(* Logix 5000 AddOnInstructionDefinition export MAC_G3_MAFR; software revision 37.00 *)

TYPE JVL_AXIS_MAC_G3 :   // Drive Data
STRUCT
   ActualMode : DINT;   // actual Mode
   ActualPosition : REAL;   // P_IST
   ActualVelocity : REAL;   // V_IST(16)
   ActualTorque : REAL;   // ACTUAL_TORQUE
   AxisStatusError : JVL_MAC_Status_Error;   // Holds an indication of which error that is detected
   Home_Mode : DINT;   // Homemode
   RequestedMode : DINT;   // requested Mode
   RequestedPosition : REAL;   // P_SOLL
   RequestedVelocity : REAL;   // V_SOLL
   RequestedAcceleration : REAL;   // A_SOLL
   GeneralCommand : DINT;
   CommandTorque : REAL;   // Requested Torque, T_SOLL
   ZeroSearchVelocity : REAL;   // Homing velocity
   ZeroSearchPosition : REAL;   // Homing position
   ZeroSearchTorque : DINT;   // Homing torque setpoint threshold value
   ZeroSearchTThreshold : DINT;   // Threshold for torque zerosearch trigger, usually 20% lower than running torque
   TravelConst : REAL;   // Factor to multiply P_IST and P_SOLL for scaling
   VelConst : REAL;   // Factor to multiply V_SOLL and V_IST to get scaled velocity value
   HomingType : DINT;   // Holds the reqested homingtype
   LoadFactor : DINT;   // Inertia ratio motor/load
   MotorType : DINT;   // MotorType configured. 0=No Selection 1=MAC50-141-A/K (old) 2=MAC50-141-F (new), MAC400, 402, 1500, 3000, 4500 (All Encoder variations) 3=MAC800 with incremental encoder 4=MAC800 with abs. encoder
   Configured : DINT;
   MSG_OutValue : DINT;   // Used in exp. output message to the motor
   MSG_InValue : DINT;   // Used in Exp. output message, to get value from motor
   MSG_OutInstance : DINT;   // Registernumber
   MSG_InInstance : DINT;   // Registernummer
   V_SOLL_CountsPerSample : REAL;
   A_SOLL_CountsPerSample2 : REAL;
   AOI_Type : DINT;   // MAC_Disable = 1, MAC_Home = 2, MAC_Jog = 3, MAC_Position = 4, MAC_Reset = 5, MAC_Stop = 6
   Position_AppType : REAL;   // calculated Position by Application Type
   MSG_Out_Execute : BOOL;   // Enable MSG_Out
   MSG_In_Execute : BOOL;   // Enable MSG_In
   ErrorReset : BOOL;
   MSG_Out_Busy : BOOL;
   MSG_In_Busy : BOOL;
   MSG_Out_Done : BOOL;
   MSG_In_Done : BOOL;
END_STRUCT
END_TYPE

TYPE JVL_MAC_Status_Error :   // Axis Faults Status
STRUCT
   Error : BOOL;
   InitialisationError : BOOL;
   FlashMemoryError : BOOL;
   STOError : BOOL;
   NotUsed_2 : BOOL;
   NotUsed_3 : BOOL;
   OUT1 : BOOL;
   OUT2 : BOOL;
   NotUsed : BOOL;
   ControlVoltageError : BOOL;
   HomingDone : BOOL;
   MotorSupplyDetected : BOOL;
   MotorLocked : BOOL;
   CommsError : BOOL;
   CurrentLoopError : BOOL;
   ModbusSlaveError : BOOL;
   TemperatureError : BOOL;
   UndervoltageError : BOOL;
   UndervoltageDetect : BOOL;
   OvervoltageError : BOOL;
   OvercurrentError : BOOL;
   OverspeedError : BOOL;
   AllowExceedingOfSoftwareLimits : BOOL;
   EncoderError : BOOL;
   I2TError : BOOL;
   FollowingError : BOOL;
   FunctionError : BOOL;
   BreakingResistorOverTempError : BOOL;
   InPosition : BOOL;
   Accelerating : BOOL;
   Decelerating : BOOL;
   SoftwareLimitExceeded : BOOL;
END_STRUCT
END_TYPE

ADD_ON_INSTRUCTION MAC_G3_MAFR   (* revision 1.0, ExecuteEnableInFalse *)
VAR_IN_OUT
   AXIS : JVL_AXIS_MAC_G3; {required}
END_VAR
VAR_OUTPUT
   EN : BOOL; {access Read Only, visible}
   CommandAborted : BOOL; {access Read Only}
   DN : BOOL; {access Read Only, visible}
   ER : BOOL; {visible}
END_VAR
VAR
   State : INT; {access None}
   ExecuteStart : BOOL; {access None}
   AOI_Type : DINT; {access None}
END_VAR

ROUTINE EnableInFalse   (* structured text *)
   State := 0;
   ExecuteStart:=0;
   	//REGION STATUS SIGNALS
   
   	    DN := State = 30;
   	    CommandAborted := State = 80;
   	    EN := EnableOut;
   	    ER:= AXIS.AxisStatusError.Error;
   	//END_REGION
   
END_ROUTINE

ROUTINE Logic   (* structured text *)
   	(*********************
   		Error Reset
   	**********************)
   
   	//REGION CAPTURE EDGES
   	    if EnableIn and not ExecuteStart then
   	    	ExecuteStart:=1;
   		//elsif not EnableIn then
   			//ExecuteStart:=0;
   		end_if;
   
   	//END_REGION
   
   	//REGION STATE CHANGES
   
   	    //Re-trigger sequence from start on rising edge
   	    //Command aborted
   	    IF AXIS.AOI_Type <> AOI_Type AND
   	        State <> 0 AND
   	        State <> 90 AND
   	        State <> 30 AND
   	        State <> 80
   	    THEN
   	        State := 80;
   	    END_IF;
   
   
   	//END_REGION
   
   	//REGION STATE MACHINE
   
   	    CASE State OF
   
   	        0:
   	            IF ExecuteStart THEN
   					AOI_Type:= 5;
   					AXIS.AOI_Type:= 5;
   	                AXIS.GeneralCommand := 16#0;
   	                State := 10;
   	            END_IF;
   
   	        10:
   	            AXIS.RequestedMode := 0;
   	            AXIS.RequestedAcceleration := 0;
   	            AXIS.RequestedPosition := 0;
   	            AXIS.RequestedVelocity := 0;
   	            AXIS.GeneralCommand := 16#10000E1;
   	            IF NOT AXIS.AxisStatusError.Error and AXIS.MotorType<>1 THEN
   	                State := 20;
   
   	            END_IF;
   
   
   	        20:
   	            AXIS.GeneralCommand := 16#0;
   	            State := 30;
   
   	        30:        //reset complete, reset to idle by setting execute false
   	            ;
   
   	        80:     //Aborted by other command before completion
   	            ;
   
   	        90:       //Error while disabling, reset to idle by setting execute false
   	            ;
   
   	        ELSE
   	            ;
   
   	    END_CASE;
   
   	//END_REGION
   
   	//REGION STATUS SIGNALS
   
   	    DN := State = 30;
   	    CommandAborted := State = 80;
   	    EN := EnableOut;
   	    ER:= AXIS.AxisStatusError.Error;
   	//END_REGION
   
END_ROUTINE
END_ADD_ON_INSTRUCTION

ADD_ON_INSTRUCTION MAC_G3_MAH   (* revision 1.0, ExecuteEnableInFalse *)
VAR_IN_OUT
   Axis : JVL_AXIS_MAC_G3; {required}
END_VAR
VAR_OUTPUT
   CommandAborted : BOOL; {access Read Only}
   EN : BOOL; {access Read Only, visible}   // Enable Bit - The EN bit stays Set until the Process is Complete and the rung goes False
   DN : BOOL; {access Read Only, visible}   // Done Bit - The Done bit is Set if the Instruction Executed without Errors
   ER : BOOL; {access Read Only, visible}   // Error Bit - An Error Happened
   IP : BOOL; {access Read Only, visible}   // In Progress Bit - The In Progress bit is Set While the Axis is Moving
   PC : BOOL; {access Read Only, visible}   // Process Complete, Motion has stopped
END_VAR
VAR_INPUT
   Mode : INT; {required}   // 0 = set Encoder, 1 = Homing on Sensor, 2 = Homing on Block
   Position : REAL; {required}   // Scaled Position after setting Encoder, with Mode = 0
   Speed : REAL; {required}   // Scaled velocity
   Acceleration : REAL; {required}   // in RPM/s
   Offset : REAL; {required}   // scaled Position after Homing, with Mode = 1 or 2
   TorqueLimit : REAL; {required}   // Homing Torque in %
END_VAR
VAR
   State : INT; {access None}
   ActiveMode : INT; {access None}
   Mode0State : INT; {access None}
   Mode1State : INT; {access None}
   Mode2State : INT; {access None}
   Mode3State : INT; {access None}
   ActivePosition : DINT; {access None}
   ActiveVelocity : DINT; {access None}
   ActiveAcceleration : REAL; {access None}
   ActiveTorqueLimit : REAL; {access None}
   ExecuteStart : BOOL; {access None}
   AOI_Type : DINT; {access None}
   ActiveDeceleration : DINT; {access None}
   Ton_wait : FBD_TIMER; {access None}
   ActiveOffset : DINT; {access None}
END_VAR

ROUTINE EnableInFalse   (* structured text *)
   State := 0;
   ExecuteStart:=0;
   	//REGION STATUS SIGNALS
   
   	    DN := State = 30;
   	    CommandAborted := State = 80;
   	    ER := State = 90;
   	    IP := State <> 0 AND NOT DN AND NOT ER AND NOT CommandAborted;
   	    EN := EnableOut;
   		PC := State = 30;
   	//END_REGION
END_ROUTINE

ROUTINE Logic   (* structured text *)
   	//REGION CAPTURE EDGES
   	    if EnableIn and not ExecuteStart then
   	    	ExecuteStart:=1;
               Axis.MSG_Out_Execute := 0;
               Axis.MSG_In_Execute := 0;
   			Ton_wait.TimerEnable:=0;
   			Ton_wait.Reset:=0;
   		elsif not EnableIn then
   			ExecuteStart:=0;
   		end_if;
   
   	//END_REGION
   	//Timer
   	TONR(Ton_wait);
   
   	//REGION STATE CHANGES
   
   	    //Re-trigger sequence from start on rising edge
   
   
   	    //Command aborted
   	    IF Axis.AOI_Type <> AOI_Type AND
   	        State <> 0 AND
   	        State <> 90 AND
   	        State <> 30 AND
   	        State <> 80
   	    THEN
   	        State := 80;
   	    END_IF;
   
   
   	    //Error if motor error while executing
   	    IF Axis.AxisStatusError.Error AND
   	        State <> 0 AND
   	        State <> 90 AND
   	        State <> 30 AND
   	        State <> 80
   	    THEN
   	        State := 90;
   	    END_IF;
   	//END_REGION
   
   	//REGION STATE MACHINE
   
   
   
   	    CASE State OF
   
   	        0:
   	            //Reset static values
   	            ActiveMode := 0;
   	            ActivePosition := 0;
   	            ActiveVelocity := 0;
   				ActiveAcceleration := 0;
   	            ActiveDeceleration := 0;
   				ActiveTorqueLimit := 0;
   	            ActiveOffset := 0;
   	            //Reset mode states
   	            Mode0State := 0;
   	            Mode1State := 0;
   	            Mode2State := 0;
   	            Mode3State := 0;
   
   	            IF ExecuteStart THEN
   					//
   					AOI_Type:= 2;
   					Axis.AOI_Type:= 2;
   	                //
   					Axis.GeneralCommand := 0;
   	                ActiveMode := Mode;
   	                ActivePosition := Position * Axis.TravelConst;
   	                ActiveVelocity := (Speed) * Axis.VelConst;// * Axis.Device.Config.V_SOLL_CountsPerSample);
   	                ActiveAcceleration := ABS(Acceleration) * Axis.A_SOLL_CountsPerSample2;
   	                //set Acceleration always >=1
   	                IF ActiveAcceleration < 1 THEN
   	                    ActiveAcceleration := 1;
   	                END_IF;
   
   	                ActiveTorqueLimit := TorqueLimit * 3.41;//1024=300%;341=100%
   	                ActiveOffset := Offset * Axis.TravelConst;
   
   
   	                State := 10;
   	            END_IF;
   
   	        10:
   	            // change to velocity mode with zero setpoint to ensure motor does not run off to current position when homed
   	            IF ActiveAcceleration < 1 THEN
   	                Axis.RequestedAcceleration := 1;
   	            ELSE
   	                Axis.RequestedAcceleration := ActiveAcceleration;
   
   	            END_IF;
   	            Axis.RequestedVelocity := 0;
   	            Axis.RequestedMode := 1;
   	            // change position setpoint to new home position
   	            Axis.RequestedPosition := ActivePosition;
   	            // reset register trigger
   	            Axis.MSG_Out_Execute := 0;
   	            Axis.MSG_In_Execute := 0;
   	            // start homing
   	            State := 20;
   
   	        20:
   	            CASE ActiveMode OF
   
   	                0:  // Set Home Position
   	                    CASE Mode0State OF
   	                        0:
   	                            if Axis.MotorType=1 then
   									Axis.MSG_OutInstance := 163;
   								else
   									Axis.MSG_OutInstance := 4;
   								end_if;
   	                            Axis.MSG_OutValue:=ActivePosition;
   	                            Axis.MSG_Out_Execute := 1;
   	                            Axis.GeneralCommand := 16#0;
   	                            IF Axis.MSG_Out_Busy AND NOT Axis.MSG_Out_Done THEN
   	                                Mode0State := 10;
   	                            END_IF;
   	                        10:
   	                            IF Axis.MSG_Out_Done THEN
   	                                Axis.MSG_Out_Execute := 0;
   	                                Mode0State := 20;
   	                            END_IF;
   	                        20:
   	                            Axis.GeneralCommand := 16#10000F7;
   	                            IF ABS(Axis.ActualPosition - ActivePosition) < 50.0 THEN
   	                                Mode0State := 30;
   	                            END_IF;
   	                        30:
   	                            Axis.GeneralCommand := 16#0;
   	                            Mode0State := 50;
   	                        50:
   	                            State := 30;
   	                        ELSE
   	                            State := 90;
   	                    END_CASE;
   
   	                1:  // Home to Sensor (type 2, bidirectional)
   	                    CASE Mode1State OF
   	                       0:
   	                            // reset hominging done bit old MAC050-141A/K
   	                                IF Axis.MotorType <> 1 THEN
   	                                    Mode1State := 10;
   	                                ELSE
   		                            Axis.MSG_OutInstance := 168;
   		                            Axis.MSG_OutValue := 0;
   		                            Axis.MSG_Out_Execute := 1;
   			                            IF Axis.MSG_Out_Busy THEN
   			                                Mode1State := 5;
   			                            END_IF;
   	                                END_IF;
   	                        5:
   	                            //Ton_Wait(IN := Reg.Done,PT := t#1s);
   	                            IF Axis.MSG_Out_Done THEN
   	                                Axis.MSG_Out_Execute := 0;
   	                                Mode1State := 10;
   	                            END_IF;
   	                       10:
   	                            //Home to Sensor (type 2);set homemode=3584
   	                            Axis.MSG_OutInstance := 42;
   	                            Axis.MSG_OutValue:=3584;
   
   	                            Axis.MSG_Out_Execute := 1;
   	                            IF Axis.MSG_Out_Busy THEN
   	                                Mode1State := 15;
   	                            END_IF;
   	                       15:
   	                            IF Axis.MSG_Out_Done THEN
   	                                Axis.MSG_Out_Execute := 0;
   	                                Mode1State := 20;
   									Axis.AxisStatusError.HomingDone:=0;
   	                            END_IF;
   
   	                       20:
   	                            // set home position offset move distance
   	                            Axis.MSG_OutInstance := 38;
   	                            Axis.MSG_OutValue:=ActiveOffset;
   	                            Axis.MSG_Out_Execute := 1;
   	                            IF Axis.MSG_Out_Busy THEN
   	                                Mode1State := 30;
   	                            END_IF;
   	                        30:
   	                            IF Axis.MSG_Out_Done THEN
   	                                Axis.MSG_Out_Execute := 0;
   	                                Mode1State := 40;
   	                            END_IF;
   	                        40:
   	                            // set homing approach velocity
   	                            Axis.MSG_OutInstance := 40;
   	                            Axis.MSG_OutValue:=ActiveVelocity;// * Axis.Device.Config.V_SOLL_CountsPerSample
   	                            Axis.MSG_Out_Execute := 1;
   	                            IF Axis.MSG_Out_Busy THEN
   	                                Mode1State := 50;
   	                            END_IF;
   	                        50:
   	                            IF Axis.MSG_Out_Done THEN
   	                                Axis.MSG_Out_Execute := 0;
   	                                Mode1State := 60;
   	                            END_IF;
   	                        60:
   	                            // start homing mode
   	                            Axis.RequestedMode := 14;
   								if Axis.MotorType=1 then
   									Axis.RequestedVelocity := ActiveVelocity;
   								end_if;
   	                            if Axis.ActualMode=14 then
   	                            	Mode1State := 70;
   	                            end_if;
   	                        70:
   	                            IF Axis.AxisStatusError.HomingDone AND Axis.MotorType <> 1 THEN
   	                                Axis.RequestedVelocity := 0;
   	                                Axis.RequestedMode := 2;
   	                                Mode1State := 80;
   	                            ELSIF Axis.Home_Mode > 0 AND Axis.MotorType = 1 THEN
   	                                Axis.RequestedVelocity := 0;
   	                                Axis.RequestedMode := 2;
   	                                Mode1State := 80;
   	                            END_IF;
   	                        80:
   	                            State := 30;
   	                        ELSE
   	                            State := 90;
   	                    END_CASE;
   
   	                2:  // Home to Endstop (torque limit)
   	                    CASE Mode2State OF
   	                        0:
   	                            //Home to Endstop (torque limit);set homemode=3072
   								Axis.MSG_OutInstance := 42;
   	                            Axis.MSG_OutValue := 3072;
   	                            Axis.MSG_Out_Execute := 1;
   
   	                            IF Axis.MSG_Out_Busy THEN
   	                                Mode2State := 5;
   	                            END_IF;
   	                        5:
   	                            IF Axis.MSG_Out_Done THEN
   	                                Axis.MSG_Out_Execute := 0;
   	                                Mode2State := 10;
   	                            END_IF;
   	                        10:
   								Axis.MSG_OutInstance := 38;
   	                            Axis.MSG_OutValue := ActiveOffset;
   	                            Axis.MSG_Out_Execute := 1;
   
   	                            IF Axis.MSG_Out_Busy THEN
   	                                Mode2State := 15;
   	                            END_IF;
   	                        15:
   	                            IF Axis.MSG_Out_Done THEN
   	                                Axis.MSG_Out_Execute := 0;
   	                                Mode2State := 20;
   									Axis.AxisStatusError.HomingDone:=0;
   	                            END_IF;
   	                        20:
   								Axis.MSG_OutInstance := 40;
   	                            Axis.MSG_OutValue := ActiveVelocity;// * Axis.Device.Config.V_SOLL_CountsPerSample;
   	                            Axis.MSG_Out_Execute := 1;
   	                            IF Axis.MSG_Out_Busy THEN
   	                                Mode2State := 25;
   	                            END_IF;
   	                        25:
   	                            IF Axis.MSG_Out_Done THEN
   	                                Axis.MSG_Out_Execute := 0;
   	                                IF Axis.MotorType <> 1 THEN
   	                                    Mode2State := 34;
   	                                ELSE
   	                                    Mode2State := 30;
   	                                END_IF;
   	                            END_IF;
   	                        30:
   	                            // reset hominging done bit old MAC050-141A/K
   								Axis.MSG_OutInstance := 168;
   	                            Axis.MSG_OutValue := 0;
   	                            Axis.MSG_Out_Execute := 1;
   
   	                            IF Axis.MSG_Out_Busy THEN
   	                                Mode2State := 32;
   	                            END_IF;
   	                        32:
   
   	                            IF Axis.MSG_Out_Done THEN
   	                                Axis.MSG_Out_Execute := 0;
   	                                Mode2State := 34;
   	                            END_IF;
   	                        34:
   								Axis.MSG_OutInstance := 41;
   	                            Axis.MSG_OutValue := ActiveTorqueLimit;
   	                            Axis.MSG_Out_Execute := 1;
   
   	                            IF Axis.MSG_Out_Busy THEN
   	                                Mode2State := 37;
   	                            END_IF;
   	                        37:
   	                            IF Axis.MSG_Out_Done THEN
   	                                Axis.MSG_Out_Execute := 0;
   	                                Mode2State := 40;
   	                            END_IF;
   	                        40:
   	                            Axis.RequestedMode := 12;
   	                            // homing done-register 42 Homemode bit 16
   								if Axis.MotorType=1 then
   									Axis.RequestedVelocity := ActiveVelocity;
   								end_if;
   	                            if Axis.ActualMode=12 then
   	                            	Mode2State := 45;
   	                            end_if;
   
   	                        45:
   	                            IF Axis.AxisStatusError.HomingDone AND Axis.MotorType <> 1 THEN
   	                                Axis.RequestedVelocity := 0;
   	                                Axis.RequestedMode := 2;
   	                                Mode2State := 60;
   	                            ELSIF Axis.Home_Mode > 0 AND Axis.MotorType = 1 THEN
   	                                Axis.RequestedVelocity := 0;
   	                                Axis.RequestedMode := 2;
   	                                Mode2State := 60;
   	                            END_IF;
   
   	                        60:
   	                            State := 30;
   	                        ELSE
   	                            State := 90;
   	                    END_CASE;
   
   
   
   	            END_CASE;
   
   	        30:        //Home complete, reset to idle by setting execute false
   	            ;
   
   	        80:     //Aborted by other command before completion
   	            ;
   
   	        90:       //Error while disabling, reset to idle by setting execute false
   	            ;
   
   	        ELSE
   	            ;
   
   	    END_CASE;
   
   	//END_REGION
   
   	//REGION STATUS SIGNALS
   
   	    DN := State = 30;
   	    CommandAborted := State = 80;
   	    ER := State = 90;
   	    IP := State <> 0 AND NOT DN AND NOT ER AND NOT CommandAborted;
   	    EN := EnableOut;
   		PC := State = 30;
   	//END_REGION
END_ROUTINE
END_ADD_ON_INSTRUCTION

ADD_ON_INSTRUCTION MAC_G3_MAJ   (* revision 1.0, ExecuteEnableInFalse *)
VAR_IN_OUT
   AXIS : JVL_AXIS_MAC_G3; {required}
END_VAR
VAR_INPUT
   Direction : DINT; {required}   // 0 = CW rotation, 1 = CCW rotation
   Speed : REAL; {required}   // scaled velocity
   Acceleration : REAL := 5000.0; {required}   // in rpm/s
END_VAR
VAR_OUTPUT
   EN : BOOL; {access Read Only, visible}   // Enable Bit - The EN bit stays Set until the Process is Complete and the rung goes False
   DN : BOOL; {access Read Only, visible}   // Done Bit - The Done bit is Set if the Instruction Executed without Errors
   ER : BOOL; {access Read Only, visible}   // Error Bit - An Error Happened
   IP : BOOL; {access Read Only, visible}   // In Progress Bit - The In Progress bit is Set While the Axis is Moving
END_VAR
VAR
   ForwardStart : BOOL; {access None}
   BackwardStart : BOOL; {access None}
   State : INT; {access None}
   ActiveVelocity : REAL; {access None}
   ActiveAcceleration : REAL; {access None}
   AOI_Type : DINT; {access None}
   ActiveDeceleration : REAL; {access None}
END_VAR

ROUTINE EnableInFalse   (* structured text *)
   	//REGION CAPTURE EDGES
   	    if Direction = 0 and EnableIn then
   	    	ForwardStart:=1;
   	    elsif Direction = 1 and EnableIn then
   	    	BackwardStart:=1;
   		elsif not EnableIn then
   	    	ForwardStart:=0;
   	    	BackwardStart:=0;
   		end_if;
   
   	//END_REGION
   
   	//REGION STATE CHANGES
   
   	    //Re-trigger sequence from start on rising edge
   	    //Command aborted
   	    IF AXIS.AOI_Type <> AOI_Type AND
   	        State <> 0 AND
   	        State <> 90 AND
   	        State <> 80
   	    THEN
   	        State := 80;
   	    END_IF;
   
   
   
   	    //Error if motor error while executing
   	    IF AXIS.AxisStatusError.Error AND
   	        State <> 0 AND
   	        State <> 90 AND
   	        State <> 80
   	    THEN
   	        State := 90;
   	    END_IF;
   
   	//END_REGION
   
   	//REGION STATE MACHINE
   
   	    CASE State OF
   
   	        0:
   	            ActiveVelocity := 0;
   	            ActiveAcceleration := 0;
   	            ActiveDeceleration := 0;
   
   	            IF ForwardStart OR BackwardStart THEN
   					DN := 0;
   					AOI_Type:= 3;
   					AXIS.AOI_Type:= 3;
   	                AXIS.RequestedMode:= 1;
   	                ActiveAcceleration := ABS(Acceleration);
   
   	                //set Acceleration always >=1
   	                IF ActiveAcceleration < 1 THEN
   	                    ActiveAcceleration := 1;
   	                END_IF;
   	                IF Direction = 0 THEN
   	                    ActiveVelocity := ABS(Speed) * AXIS.VelConst;// * Axis.Device.Config.V_SOLL_CountsPerSample));
   	                    State := 10;
   	                ELSIF Direction = 1 THEN
   	                    ActiveVelocity := -1.0 * ABS(Speed)* AXIS.VelConst;// * Axis.Device.Config.V_SOLL_CountsPerSample));
   	                    State := 10;
   	                ELSE
   	                    State := 30;
   	                END_IF;
   
   	                State := 10;
   	            END_IF;
   
   	        10:
   	            IF AXIS.ActualMode = 1 THEN
   
   	                AXIS.RequestedAcceleration := ActiveAcceleration;
   	                AXIS.RequestedVelocity := ActiveVelocity;
                       State := 30;
   
   	            END_IF;
   
   	        20:
   	            IF AXIS.ActualMode = 1 THEN
   
   	                IF not EnableIn THEN
   	                    State := 30;
   	                END_IF;
   
   	            ELSE
   	                State := 80;
   	            END_IF;
   
   
   	        30:
   	            AXIS.RequestedMode := 1;
   	            AXIS.RequestedVelocity := 0;
   
   	            State := 40;
   
   	        40:
   	            IF AXIS.ActualMode = 1  THEN
   
   	                //If no motion then stop is complete
   	                IF ABS((AXIS.ActualVelocity)) <= 10.0 AND
   	                    NOT AXIS.AxisStatusError.Accelerating AND
   	                    NOT AXIS.AxisStatusError.Decelerating THEN
   	                    State := 0;
   						DN := 1;
   	                END_IF;
   
   	            ELSE
   	                State := 80;
   	            END_IF;
   
   	        80:     //Aborted by other command before completion
   	            IF NOT EnableIn THEN
   	                State := 0;
   	            END_IF;
   
   	        90:       //Error while jogging, reset to idle by setting jog inputs false
   	            IF NOT EnableIn THEN
   	                State := 0;
   	            END_IF;
   
   	        ELSE
   	            State := 90;
   
   	    END_CASE;
   
   	//END_REGION
   
   	//REGION STATUS SIGNALS
   
   	    EN:=EnableOut;
   						//(State=20 or State = 25) AND
   	                    //  AXIS.AxisStatus.AtVelocity AND
   	                    //  NOT AXIS.AxisStatus.Accelerating AND
   	                    //  NOT AXIS.AxisStatus.Decelerating;
   	    DN := State = 40;
   	    ER := State = 90;
   	    IP := State <> 0 AND NOT ER AND NOT DN;
   
   	//END_REGION
   
END_ROUTINE

ROUTINE Logic   (* structured text *)
   	//REGION CAPTURE EDGES
   	    if Direction = 0 and EnableIn then
   	    	ForwardStart:=1;
   	    elsif Direction = 1 and EnableIn then
   	    	BackwardStart:=1;
   		elsif not EnableIn then
   	    	ForwardStart:=0;
   	    	BackwardStart:=0;
   		end_if;
   
   	//END_REGION
   
   	//REGION STATE CHANGES
   
   	    //Re-trigger sequence from start on rising edge
   	    //Command aborted
   	    IF AXIS.AOI_Type <> AOI_Type AND
   	        State <> 0 AND
   	        State <> 90 AND
   	        State <> 80
   	    THEN
   	        State := 80;
   	    END_IF;
   
   
   
   	    //Error if motor error while executing
   	    IF AXIS.AxisStatusError.Error AND
   	        State <> 0 AND
   	        State <> 90 AND
   	        State <> 80
   	    THEN
   	        State := 90;
   	    END_IF;
   
   	//END_REGION
   
   	//REGION STATE MACHINE
   
   	    CASE State OF
   
   	        0:
   	            ActiveVelocity := 0;
   	            ActiveAcceleration := 0;
   	            ActiveDeceleration := 0;
   
   	            IF ForwardStart OR BackwardStart THEN
   					DN := 0;
   					AOI_Type:= 3;
   					AXIS.AOI_Type:= 3;
   	                AXIS.RequestedMode:= 1;
   	                ActiveAcceleration := ABS(Acceleration)* AXIS.A_SOLL_CountsPerSample2;
   	                //set Acceleration always >=1
   	                IF ActiveAcceleration < 1 THEN
   	                    ActiveAcceleration := 1;
   	                END_IF;
   	                IF Direction = 0 THEN
   	                    ActiveVelocity := ABS(Speed) * AXIS.VelConst;// * Axis.Device.Config.V_SOLL_CountsPerSample));
   	                    State := 10;
   	                ELSIF Direction = 1 THEN
   	                    ActiveVelocity := -1.0 * ABS(Speed)* AXIS.VelConst;// * Axis.Device.Config.V_SOLL_CountsPerSample));
   	                    State := 10;
   	                ELSE
   	                    State := 30;
   	                END_IF;
   
   	                State := 10;
   	            END_IF;
   
   	        10:
   	            IF AXIS.ActualMode = 1 THEN
   
   	                AXIS.RequestedAcceleration := ActiveAcceleration;
   	                AXIS.RequestedVelocity := ActiveVelocity;
   	                IF not EnableIn THEN
   	                    State := 30;
   	                END_IF;
   
   	            END_IF;
   
   	        20:
   	            IF AXIS.ActualMode = 1 THEN
   
   	                IF not EnableIn THEN
   	                    State := 30;
   	                END_IF;
   
   	            ELSE
   	                State := 80;
   	            END_IF;
   
   
   	        30:
   	            AXIS.RequestedMode := 1;
   	            AXIS.RequestedVelocity := 0;
   
   	            State := 40;
   
   	        40:
   	            IF AXIS.ActualMode = 1  THEN
   
   	                //If no motion then stop is complete
   	                IF ABS((AXIS.ActualVelocity)) <= 10.0 AND
   	                    NOT AXIS.AxisStatusError.Accelerating AND
   	                    NOT AXIS.AxisStatusError.Decelerating THEN
   	                    State := 0;
   						DN := 1;
   	                END_IF;
   
   	            ELSE
   	                State := 80;
   	            END_IF;
   
   	        80:     //Aborted by other command before completion
   	            IF NOT EnableIn THEN
   	                State := 0;
   	            END_IF;
   
   	        90:       //Error while jogging, reset to idle by setting jog inputs false
   	            IF NOT EnableIn THEN
   	                State := 0;
   	            END_IF;
   
   	        ELSE
   	            State := 90;
   
   	    END_CASE;
   
   	//END_REGION
   
   	//REGION STATUS SIGNALS
   
   	    EN:=EnableOut;
   						//(State=20 or State = 25) AND
   	                    //  AXIS.AxisStatus.AtVelocity AND
   	                    //  NOT AXIS.AxisStatus.Accelerating AND
   	                    //  NOT AXIS.AxisStatus.Decelerating;
   	    DN := State = 40;
   	    ER := State = 90;
   	    IP := State <> 0 AND NOT ER AND NOT DN;
   
   	//END_REGION
   
END_ROUTINE
END_ADD_ON_INSTRUCTION

ADD_ON_INSTRUCTION MAC_G3_MAM   (* revision 1.0, ExecuteEnableInFalse *)
VAR_IN_OUT
   Axis : JVL_AXIS_MAC_G3; {required}
END_VAR
VAR_INPUT
   MoveType : DINT; {required}   // 0=absolute, 1= relative
   Position : REAL; {required}   // scaled Position
   Speed : REAL; {required}   // scaled velocity
   Acceleration : REAL; {required}   // in rpm/s
END_VAR
VAR_OUTPUT
   CommandAborted : BOOL; {access Read Only}
   EN : BOOL; {visible}   // Enable Bit - The EN bit stays Set until the Process is Complete and the rung goes False
   DN : BOOL; {access Read Only, visible}   // Done Bit - The Done bit is Set if the Instruction Executed without Errors
   ER : BOOL; {access Read Only, visible}   // Error Bit - An Error Happened
   IP : BOOL; {access Read Only, visible}   // In Progress Bit - The In Progress bit is Set While the Axis is Moving
   PC : BOOL; {visible}   // Process Complete, Motion has stopped
END_VAR
VAR
   State : INT; {access None}
   ExecuteStart : BOOL; {access None}
   ActiveAbsolute : BOOL; {access None}
   ActiveVelocity : DINT; {access None}
   ActiveAcceleration : REAL; {access None}
   ActiveTargetPosition : DINT; {access None}
   StartPosition : REAL; {access None}
   AOI_Type : DINT; {access None}
END_VAR

ROUTINE EnableInFalse   (* structured text *)
   State := 0;
   ExecuteStart:=0;
   	    DN := State = 30 OR State = 35;
   		PC:= State = 30 OR State = 35;
   	    CommandAborted := State = 80;
   	    ER := State = 90;
   	    IP := State <> 0 AND NOT DN AND NOT ER AND NOT CommandAborted;
   	    EN:= EnableOut;
   
END_ROUTINE

ROUTINE Logic   (* structured text *)
   	//REGION CAPTURE EDGES
   	    if EnableIn and not ExecuteStart then
   	    	ExecuteStart:=1;
   			State:= 0;
   
   		end_if;
   
   	//END_REGION
   
   	//REGION STATE CHANGES
   
   	    //Re-trigger sequence from start on rising edge
   
   
   	    //Command aborted
   	    IF Axis.AOI_Type <> AOI_Type AND
   	        State <> 0 AND
   	        State <> 90 AND
   	        State <> 30 AND
   	        State <> 80
   	    THEN
   	        State := 80;
   	    END_IF;
   
   
   	    //Error if motor error while executing
   	    IF Axis.AxisStatusError.Error AND
   	        State <> 0 AND
   	        State <> 90 AND
   	        State <> 30 AND
   	        State <> 80
   	    THEN
   	        State := 90;
   	    END_IF;
   	//END_REGION
   
   	//REGION STATE MACHINE
   
   	    CASE State OF
   
   	        0:
   	            ActiveVelocity := 0;
   	            ActiveAcceleration := 0;
   				ActiveAbsolute := 0;
   	            ActiveTargetPosition := 0;
   
   	            IF ExecuteStart THEN
   					AOI_Type:= 4;
   					Axis.AOI_Type:= 4;
   	                Axis.RequestedMode := 2;
   	                StartPosition := Axis.ActualPosition;// *Axis.TravelConst;
   	                ActiveVelocity := ABS(Speed) * Axis.VelConst;// * Axis.Device.Config.V_SOLL_CountsPerSample);
   	                ActiveAcceleration := ABS(Acceleration)* Axis.A_SOLL_CountsPerSample2;
   	                //set Acceleration always >=1
   	                IF ActiveAcceleration < 1.0 THEN
   	                    ActiveAcceleration := 1.0;
   	                END_IF;
   
   					if MoveType= 0 then
   	                	ActiveAbsolute := 1;
   					elsif MoveType = 1 then
   						ActiveAbsolute:= 0;
   					end_if;
   
   
   
   	                IF ActiveAbsolute THEN
   	                    ActiveTargetPosition := Position *Axis.TravelConst;
   	                ELSE
   	                    ActiveTargetPosition := Position *Axis.TravelConst+ StartPosition;
   	                END_IF;
   
   	                State := 10;
   	            END_IF;
   
   	        10:
   	            IF Axis.ActualMode = 2 THEN
   	                Axis.RequestedAcceleration := ActiveAcceleration;
   	                Axis.RequestedPosition := ActiveTargetPosition;
   	                Axis.RequestedVelocity := ActiveVelocity;
   
   					State := 20;
   					(*
   	                IF ContinuousUpdate THEN
   	                    State := 25;
   	                ELSE
   	                    State := 20;
   	                END_IF;
   	                *)
   	            END_IF;
   
   	        20:
   	            IF Axis.ActualMode = 2 AND
   	                Axis.RequestedPosition = ActiveTargetPosition AND
   	                Axis.RequestedVelocity = ActiveVelocity THEN
   
   	                //If taget reached then move is complete
   	                IF ABS(ActiveTargetPosition - Axis.ActualPosition) <= 10 AND
   	                    Axis.AxisStatusError.InPosition AND
   	                    NOT Axis.AxisStatusError.Accelerating AND
   	                    NOT Axis.AxisStatusError.Decelerating THEN
   	                    State := 30;
   	                END_IF;
   
   	            ELSE
   	                State := 80;
   	            END_IF;
   
   	        30:
   	            ;
   	        (*
   	        25:
   	            IF Axis.Telegram.Input.OperatingMode = 2 AND
   	                Axis.Telegram.Output.VelocitySetpoint = DINT_TO_DWORD(ActiveVelocity) AND
   	                Axis.Telegram.Output.PositionSetpoint = DINT_TO_DWORD(ActiveTargetPosition) THEN
   
   	                IF Execute THEN
   
   	                    ActiveVelocity := LREAL_TO_DINT(ABS(Velocity) * Axis.Device.Config.V_SOLL_CountsPerSample);
   	                    ActiveAcceleration := LREAL_TO_DINT(ABS(Acceleration) * Axis.Device.Config.A_SOLL_CountsPerSample2);
   	                    //set Acceleration always >=1
   	                    IF ActiveAcceleration < 1 THEN
   	                        ActiveAcceleration := 1;
   	                    END_IF;
   	                    IF ActiveAbsolute THEN
   	                        ActiveTargetPosition := Position;
   	                    ELSE
   	                        ActiveTargetPosition := Position + StartPosition;
   	                    END_IF;
   
   	                    Axis.Telegram.Output.AccelerationSetpoint := ActiveAcceleration;
   	                    Axis.Telegram.Output.PositionSetpoint := ActiveTargetPosition;
   	                    Axis.Telegram.Output.VelocitySetpoint := ActiveVelocity;
   
   	                    //If taget reached then move is complete
   	                    IF ABS(DINT_TO_LREAL(ActiveTargetPosition - Axis.Telegram.Input.ActualPosition)) <= 5.0 AND
   	                        Axis.Telegram.Input.StatusError.InPosition AND
   	                        NOT Axis.Telegram.Input.StatusError.Accelerating AND
   	                        NOT Axis.Telegram.Input.StatusError.Decelerating THEN
   	                        State := 35;
   	                    END_IF;
   
   	                ELSE
   	                    State := 20;
   	                END_IF;
   
   	            ELSE
   	                State := 80;
   	            END_IF;
   
   	        35:
   	            IF Execute THEN
   
   	                IF ActiveAbsolute THEN
   	                    IF ActiveTargetPosition <> Position THEN
   	                        State := 20;
   	                    END_IF;
   	                ELSE
   	                    IF ActiveTargetPosition <> (Position + StartPosition) THEN
   	                        State := 25;
   	                    END_IF;
   	                END_IF;
   
   	            ELSE
   	                State := 0;
   	            END_IF;
   	        *)
   	        80:     //Aborted by other command before completion
   	           ;
   
   	        90:       //Error, reset to idle by setting execute false
   	            ;
   	            //Mode=Passiv
   	            Axis.RequestedMode := 0;
   	        ELSE
   	            ;
   
   	    END_CASE;
   
   	//END_REGION
   
   	//REGION STATUS SIGNALS
   
   	    DN := State = 30 OR State = 35;
   		PC:= State = 30 OR State = 35;
   	    CommandAborted := State = 80;
   	    ER := State = 90;
   	    IP := State <> 0 AND NOT DN AND NOT ER AND NOT CommandAborted;
   	    EN:= EnableOut;
   	//END_REGION
END_ROUTINE
END_ADD_ON_INSTRUCTION

ADD_ON_INSTRUCTION MAC_G3_MAS   (* revision 1.0, ExecuteEnableInFalse *)
VAR_IN_OUT
   AXIS : JVL_AXIS_MAC_G3; {required}
END_VAR
VAR_INPUT
   Decel_Rate : REAL; {required}   // in RPM/s
END_VAR
VAR_OUTPUT
   CommandAborted : BOOL; {access Read Only}
   EN : BOOL; {access Read Only, visible}
   DN : BOOL; {access Read Only, visible}
   ER : BOOL; {access Read Only, visible}
   IP : BOOL; {access Read Only, visible}
   PC : BOOL; {access Read Only, visible}
END_VAR
VAR
   State : INT; {access None}
   ExecuteStart : BOOL; {access None}
   ActiveDeceleration : DINT; {access None}
   AOI_Type : DINT; {access None}
END_VAR

ROUTINE EnableInFalse   (* structured text *)
   State := 0;
   ExecuteStart:=0;
   
   	    DN := State = 30;
   	    CommandAborted := State = 80;
   	    ER := State = 90;
   	    IP := State<> 0 AND NOT DN AND NOT ER AND NOT CommandAborted;
   	    EN:=EnableOut;
   		PC := State = 30;
   
END_ROUTINE

ROUTINE Logic   (* structured text *)
   	//REGION CAPTURE EDGES
   	    if EnableIn and not ExecuteStart then
   	    	ExecuteStart:=1;
   
   		end_if;
   
   	//END_REGION
   
   	//REGION STATE CHANGES
   
   	    //Re-trigger sequence from start on rising edge
   
   	    //Command aborted
   	    IF AXIS.AOI_Type <> AOI_Type AND
   	        State <> 0 AND
   	        State <> 90 AND
   	        State <> 30 AND
   	        State <> 80
   	    THEN
   	        State := 80;
   	    END_IF;
   
   	    //Error if motor error while executing
   	    IF AXIS.AxisStatusError.Error AND
   	        State <> 0 AND
   	        State <> 90 AND
   	        State <> 30 AND
   	        State <> 80
   	    THEN
   	        State := 90;
   	    END_IF;
   
   	//END_REGION
   
   	//REGION STATE MACHINE
   
   	    CASE State OF
   
   	        0:        //Wait for rising edge on execute
   	            ActiveDeceleration := 0;
   
   	            IF ExecuteStart THEN
   					AOI_Type:= 6;
   					AXIS.AOI_Type:= 6;
   	                AXIS.RequestedMode:= 1;
   	                ActiveDeceleration :=  Decel_Rate;//
   	                //set Acceleration always >=1
   	                IF ActiveDeceleration < 1 THEN
   	                    ActiveDeceleration := 1;
   	                END_IF;
   	                State := 10;
   	            END_IF;
   
   	        10:        //Trigger stop
   	            IF AXIS.ActualMode = 1 THEN
   	                AXIS.RequestedAcceleration := ActiveDeceleration;
   	                AXIS.RequestedVelocity := 0;
   	                State := 20;
   
   	            ELSE            //Go to Idle if other command has changed the operating state
   	                State := 0;
   	            END_IF;
   
   	        20:    //Check stop is complete
   	            IF AXIS.RequestedMode = 1 AND
   	                AXIS.RequestedVelocity = 0 THEN
   
   	                //If no motion then stop is complete
   	                IF ABS(AXIS.ActualVelocity) <= 10.0 AND
   	                    NOT AXIS.AxisStatusError.Accelerating and
   	                    NOT AXIS.AxisStatusError.Decelerating THEN
   	                    State := 30;
   	                END_IF;
   
   	            ELSE            //Go to Idle if other command has changed the operating state
   	                State := 0;
   	            END_IF;
   
   	        30:        //Disable complete, reset to idle by setting execute false
   	            IF NOT EnableIn THEN
   	                ;
   	            END_IF;
   
   	        80:     //Aborted by other command before completion
   	            IF NOT EnableIn THEN
   					;
   				END_IF;
   
   	        90:       //Error while disabling, reset to idle by setting execute false
   	            IF NOT EnableIn THEN
   	                ;
   	            END_IF;
   
   	        ELSE
   	            ;
   
   	    END_CASE;
   
   	//END_REGION
   
   	//REGION STATUS SIGNALS
   
   	    DN := State = 30;
   	    CommandAborted := State = 80;
   	    ER := State = 90;
   	    IP := State<> 0 AND NOT DN AND NOT ER AND NOT CommandAborted;
   	    EN:=EnableOut;
   		PC := State = 30;
   
   	//END_REGION
END_ROUTINE
END_ADD_ON_INSTRUCTION

ADD_ON_INSTRUCTION MAC_G3_MSF   (* revision 1.0, ExecuteEnableInFalse *)
VAR_IN_OUT
   AXIS : JVL_AXIS_MAC_G3; {required}
END_VAR
VAR_OUTPUT
   EN : BOOL; {access Read Only, visible}
   CommandAborted : BOOL; {access Read Only}
   DN : BOOL; {access Read Only, visible}
   ER : BOOL; {access Read Only, visible}
END_VAR
VAR
   State : INT; {access None}
   ExecuteStart : BOOL; {access None}
   AOI_Type : DINT; {access None}
END_VAR

ROUTINE EnableInFalse   (* structured text *)
   State := 0;
   ExecuteStart:=0;
   	//REGION STATUS SIGNALS
   
   	    DN := State = 20;
   	    CommandAborted := State = 80;
   	    ER := State = 90;
   	    EN := EnableOut;
   
   	//END_REGION
   
END_ROUTINE

ROUTINE Logic   (* structured text *)
   	///REGION CAPTURE EDGES
   
   	 	if EnableIn and not ExecuteStart then
   	    	ExecuteStart:=1;
   		end_if;
   	///END_REGION
   
   	//REGION STATE CHANGES
   
   	    //Re-trigger sequence from start on rising edge
   
   	    //Command aborted
   	    IF AXIS.AOI_Type <> AOI_Type AND
   	        State <> 0 AND
   	        State <> 90 AND
   	        State <> 30 AND
   	        State <> 80
   	    THEN
   	        State := 80;
   	    END_IF;
   
   
   	    //Error if motor error while executing
   	    IF AXIS.AxisStatusError.Error AND
   	        State <> 0 AND
   	        State <> 90 AND
   	        State <> 20 AND
   	        State <> 80
   	    THEN
   	        State := 90;
   	    END_IF;
   
   	//END_REGION
   
   	//REGION STATE MACHINE
   
   	    CASE State OF
   
   	        0:        //Wait for rising edge on execute
   	            IF ExecuteStart THEN
   					AOI_Type:= 1;
   					AXIS.AOI_Type:= 1;
   	                State := 10;
   	            END_IF;
   
   	        10:     //Put JVL into passive state
   	            AXIS.RequestedMode:= 0;
   	            IF AXIS.ActualMode = 0 THEN
   	                State := 20;
   	            END_IF;
   
   	        20:        //Disable complete, reset to idle by setting execute false
   	            ;
   
   	        80:     //Aborted by other command before completion
   	            ;
   
   	        90:       //Error while disabling, reset to idle by setting execute false
   	           ;
   
   	        ELSE
   	            ;//State := 90;
   
   	    END_CASE;
   
   	//END_REGION
   
   	//REGION STATUS SIGNALS
   
   	    DN := State = 20;
   	    CommandAborted := State = 80;
   	    ER := State = 90;
   	    EN := EnableOut;
   
   	//END_REGION
   
END_ROUTINE
END_ADD_ON_INSTRUCTION
